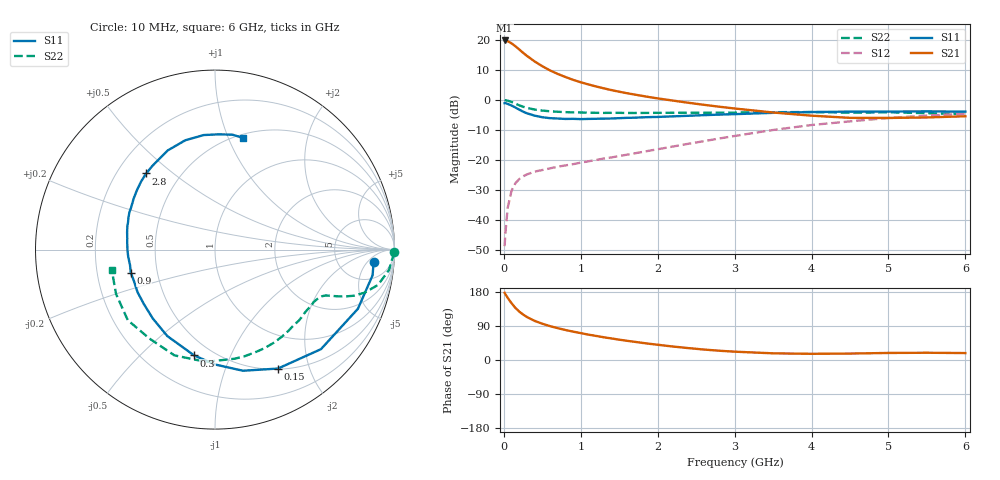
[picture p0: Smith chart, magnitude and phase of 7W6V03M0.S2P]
! Infineon Technologies  Discrete & RF Semiconductors
! BFS17W
! Si NPN RF Bipolar Junction Transistor in SOT323
! VCE = 6 V  IC = 3 mA
! Common Emitter S-Parameters:  August  1999
# GHz  S  MA  R  50
!  f  S11  S21  S12  S22
! GHz  MAG  ANG  MAG  ANG  MAG  ANG  MAG  ANG
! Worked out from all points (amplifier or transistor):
!   36 points, 10 MHz to 6 GHz, reference 50 ohm
!   highest |S21| = 19.8 dB at 10 MHz (marker M1)
!   |S21| within 3 dB of that: start of sweep to 200.5 MHz
!   unconditionally stable (mu >= 1): 730.5 MHz to 2.697 GHz; 4.438 GHz to end of sweep
!   at 250 MHz: K = 0.44, MSG = 20.6 dB, |S12| = -25.4 dB
!   at 1.4 GHz: K = 1.26, MAG = 8.2 dB, |S12| = -19.1 dB
!   at 6 GHz: K = 1.07, MAG = -2.1 dB, |S12| = -4.5 dB
!   S11 on the Smith chart (normalised r, x): 10 MHz: 12, -8; 150 MHz: 0.51, -1.54; 300 MHz: 0.40, -0.74; 900 MHz: 0.35, -0.12; 2.8 GHz: 0.32, +0.41; 6 GHz: 0.53, +1.13
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0.01  0.8867 -4.5  9.801 177.3  0.0037 90.1  0.9986 -0.9
0.02  0.8895 -9.3  9.774 173.6  0.006 81.9  0.9897 -2.8
0.05  0.8618 -22.5  9.53 164.0  0.0161 80.2  0.976 -6.7
0.1  0.8101 -43.2  8.769 150.0  0.0309 68.1  0.9296 -12.2
0.15  0.7499 -62.1  7.858 137.5  0.0413 59.8  0.8685 -16.0
0.2  0.6927 -77.0  6.948 127.9  0.0484 54.9  0.8175 -18.3
0.25  0.6403 -89.9  6.118 120.0  0.0537 50.4  0.7736 -19.7
0.3  0.6012 -101.1  5.432 113.5  0.0578 48.3  0.741 -20.6
0.4  0.5501 -118.9  4.386 103.3  0.0644 45.8  0.6939 -21.8
0.5  0.5171 -132.1  3.652 95.7  0.0685 45.3  0.6672 -22.5
0.6  0.4992 -142.5  3.109 89.4  0.0729 46.1  0.6495 -23.6
0.7  0.4925 -151.2  2.72 84.0  0.0777 48.0  0.6379 -24.9
0.9  0.4865 -164.6  2.169 74.9  0.0857 50.5  0.6226 -28.0
1.1  0.4852 -175.3  1.817 66.9  0.0956 54.0  0.6162 -31.8
1.3  0.4905 175.8  1.565 60.0  0.1064 57.3  0.6108 -36.1
1.6  0.5052 165.2  1.298 50.7  0.123 61.2  0.6088 -42.8
2.2  0.5352 147.8  0.978 35.5  0.1686 67.0  0.6136 -57.9
2.8  0.5717 132.1  0.774 24.5  0.2289 68.4  0.6165 -74.5
3.5  0.612 115.5  0.62 17.6  0.3175 65.2  0.6276 -94.6
4.5  0.6413 95.6  0.505 17.0  0.4414 53.6  0.6155 -126.5
5.5  0.6475 81.3  0.513 19.1  0.5504 40.3  0.6043 -155.8
6  0.6417 76.0  0.537 18.3  0.5924 33.8  0.5862 -168.8
